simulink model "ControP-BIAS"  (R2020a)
settings: Solver=ode45  StartTime=0.0  StopTime=30  RelTol=1e-3  EnableMultiTasking=on
libraries: simulink x5

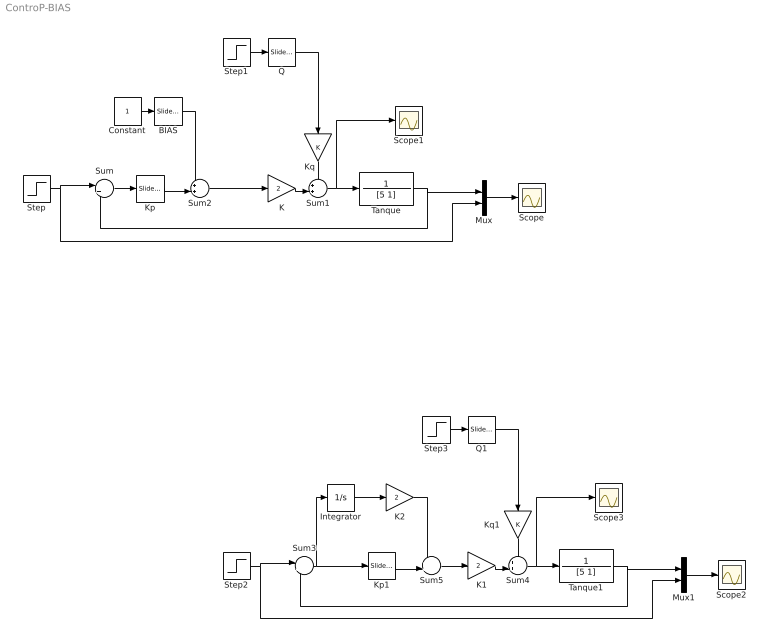
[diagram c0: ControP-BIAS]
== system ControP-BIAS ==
  BIAS : simulink/Math Operations/Slider Gain  gain=0.275  low=0  high=1
  Constant : Constant
  Integrator : Integrator
  K : Gain  Gain=2
  K1 : Gain  Gain=2
  K2 : Gain  Gain=2
  Kp : simulink/Math Operations/Slider Gain  gain=2.0  low=0  high=20
  Kp1 : simulink/Math Operations/Slider Gain  gain=2.0  low=0  high=20
  Kq : Gain
  Kq1 : Gain
  Mux : Mux  Inputs=2
  Mux1 : Mux  Inputs=2
  Q : simulink/Math Operations/Slider Gain  gain=0.450  low=0  high=1
  Q1 : simulink/Math Operations/Slider Gain  gain=0.450  low=0  high=1
  Scope{,1..3} (4 alike) : Scope
  Step : Step  Time=0  SampleTime=0
  Step1 : Step  Time=20
  Step2 : Step  Time=0  SampleTime=0
  Step3 : Step  Time=20
  Sum : Sum  Inputs=|+-
  Sum{1..2,4..5} (4 alike) : Sum  Inputs=++|
  Sum3 : Sum  Inputs=|+-
  Tanque : TransferFcn  Numerator=1  Denominator=[5 1]
  Tanque1 : TransferFcn  Numerator=1  Denominator=[5 1]
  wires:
  Sum/1 -> Kp/1
  Mux/1 -> Scope/1
  Step/1 -> Mux/2, Sum/1
  Sum1/1 -> Scope1/1, Tanque/1
  K/1 -> Sum1/2
  Kq/1 -> Sum1/1
  Kp/1 -> Sum2/2
  Constant/1 -> BIAS/1
  BIAS/1 -> Sum2/1
  Step1/1 -> Q/1
  Q/1 -> Kq/1
  Sum2/1 -> K/1
  Tanque/1 -> Sum/2, Mux/1
  Q1/1 -> Kq1/1
  Step3/1 -> Q1/1
  Mux1/1 -> Scope2/1
  Sum4/1 -> Scope3/1, Tanque1/1
  K1/1 -> Sum4/2
  Tanque1/1 -> Sum3/2, Mux1/1
  Step2/1 -> Mux1/2, Sum3/1
  Kq1/1 -> Sum4/1
  Integrator/1 -> K2/1
  Sum3/1 -> Kp1/1, Integrator/1
  Sum5/1 -> K1/1
  Kp1/1 -> Sum5/2
  K2/1 -> Sum5/1
